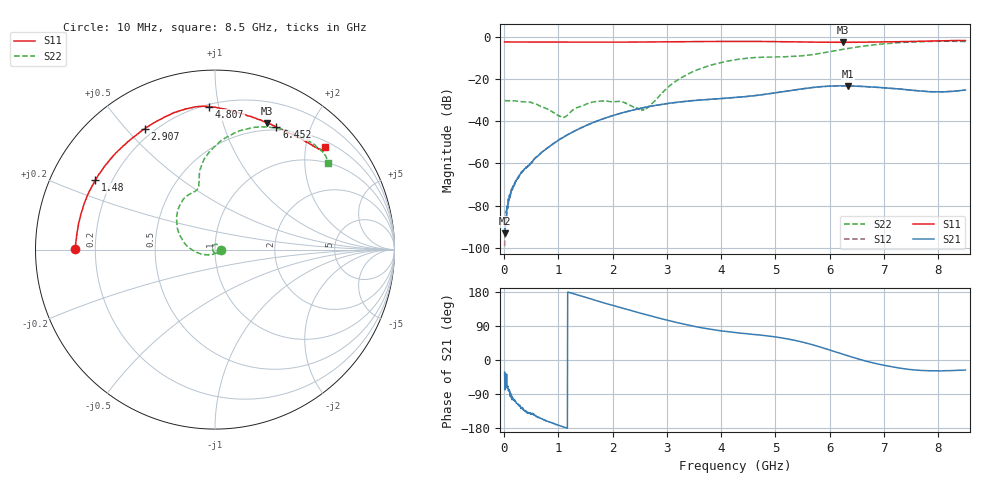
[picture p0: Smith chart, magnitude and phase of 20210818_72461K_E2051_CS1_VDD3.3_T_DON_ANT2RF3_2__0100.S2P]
!Agilent Technologies,E5071C,MY46417908,A.11.23
!Date: Wed Aug 18 14:29:26 2021
!Data & Calibration Information:
!Freq	S11:SOLT2(ON)	S21:SOLT2(ON)	S12:SOLT2(ON)	S22:SOLT2(ON)
!PortZ  Port1:50+j0  Port2:50+j0
!Above PortZ is port z conversion or system Z0 setting when saving the data.
!When reading, reference impedance value at option line is always used.
# Hz S dB R 50
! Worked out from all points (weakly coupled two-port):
!   1601 points, 10 MHz to 8.5 GHz, reference 50 ohm
!   highest |S21| = -23.06 dB at 6.34 GHz (marker M1); lowest = -93.2 dB at 15.31 MHz (marker M2)
!   lowest |S11| = -2.4 dB at 6.25 GHz (marker M3), VSWR 7.37, Z = 21.1 + j70.5 ohm
!   |S11| at or under -10 dB: nowhere
!   |S22| runs from -38.1 to -1.8 dB; largest |S21 - S12| = 0.00032
!   S11 on the Smith chart (normalised r, x): 10 MHz: 0.12, +0.00; 1.48 GHz: 0.14, +0.26; 2.907 GHz: 0.16, +0.56; 4.807 GHz: 0.22, +0.94; 6.452 GHz: 0.47, +1.52; 8.5 GHz: 0.62, +2.40
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1e7  -2.15 179.7  -89.78 -32.6  -99.32 94.7  -29.92 -2.1
1.530625e7  -2.17 179.6  -93.19 -79.0  -92.64 -76.0  -29.98 -2.5
6.836875e7  -2.19 178.5  -79.56 -68.4  -80.01 -74.9  -30.15 -6.2
2.647e8  -2.21 174.4  -66.64 -118.9  -66.42 -116.2  -30.43 -24.0
5.724625e8  -2.24 168.2  -57.44 -147.1  -57.52 -146.4  -31.53 -60.6
1.081862e9  -2.25 157.9  -47.61 -176.2  -47.66 -176.2  -37.92 -165.9
1.426769e9  -2.26 151.0  -42.93 168.5  -42.96 168.5  -32.77 117.9
1.479831e9  -2.26 149.9  -42.30 166.3  -42.31 166.4  -32.19 109.2
2.1325e9  -2.26 136.4  -36.23 138.9  -36.25 138.8  -30.51 29.0
2.557e9  -2.24 127.4  -33.49 122.0  -33.49 121.9  -34.26 -55.1
2.843538e9  -2.18 121.4  -32.14 110.9  -32.14 110.7  -28.27 -133.2
2.907212e9  -2.17 120.2  -31.92 108.7  -31.92 108.6  -26.73 -142.8
3.464369e9  -2.03 110.1  -30.13 90.1  -30.12 90.1  -16.46 174.5
4.255e9  -1.92 98.8  -28.62 72.3  -28.62 72.3  -10.68 136.1
4.80685e9  -1.98 92.3  -27.09 64.4  -27.09 64.4  -9.42 116.6
5.671769e9  -2.23 79.1  -23.91 40.7  -23.91 40.8  -8.26 103.4
6.25015e9  -2.37 67.6  -23.08 14.9  -23.10 14.9  -5.69 95.7
6.340356e9  -2.33 65.6  -23.06 10.8  -23.08 10.8  -5.28 93.4
6.451788e9  -2.35 63.3  -23.18 5.9  -23.20 5.7  -4.82 90.2
7.088538e9  -2.11 51.3  -24.17 -16.4  -24.20 -16.6  -2.85 71.3
7.937538e9  -1.67 42.3  -25.89 -28.4  -25.86 -28.5  -1.88 46.5
8.5e9  -1.53 43.0  -25.10 -26.7  -25.09 -27.0  -2.03 37.3
